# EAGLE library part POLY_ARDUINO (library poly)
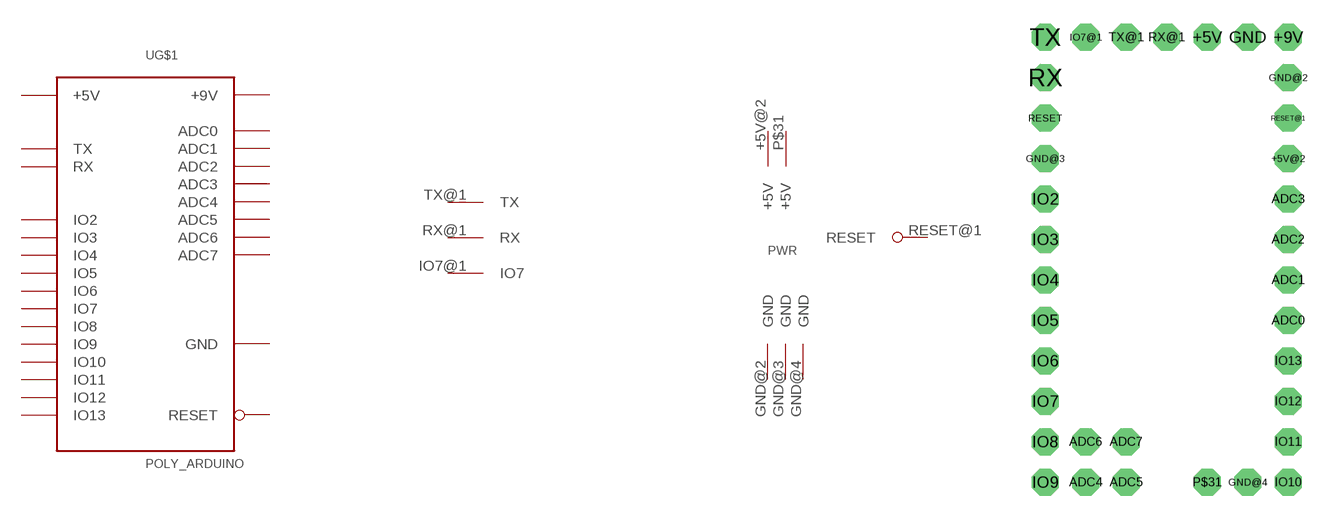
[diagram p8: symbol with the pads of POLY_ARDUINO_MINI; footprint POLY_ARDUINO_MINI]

Designator prefix -; gates G$1=POLY_ARDUINO G$2=POLY_ARDUINO_MINI_GND G$3=POLY_ARDUINO_MINI_OPT_IO

## POLY_ARDUINO  [POLY_ARDUINO_MINI]
+5V  G$1:+5V  pwr
+5V@2  G$2:+5V  pwr
+9V  G$1:+9V  pwr
ADC0  G$1:ADC0  in
ADC1  G$1:ADC1  in
ADC2  G$1:ADC2  in
ADC3  G$1:ADC3  in
ADC4  G$1:ADC4  in
ADC5  G$1:ADC5  in
ADC6  G$1:ADC6  in
ADC7  G$1:ADC7  in
GND  G$1:GND  sup
GND@2  G$2:GND  pwr
GND@3  G$2:GND  pwr
GND@4  G$2:GND  pwr
IO2  G$1:IO2
IO3  G$1:IO3
IO4  G$1:IO4
IO5  G$1:IO5
IO6  G$1:IO6
IO7  G$1:IO7
IO7@1  G$3:IO7
IO8  G$1:IO8
IO9  G$1:IO9
IO10  G$1:IO10
IO11  G$1:IO11
IO12  G$1:IO12
IO13  G$1:IO13
P$31  G$2:+5V  pwr
RESET  G$1:RESET
RESET@1  G$2:RESET  in
RX  G$1:RX  in
RX@1  G$3:RX  in
TX  G$1:TX  out
TX@1  G$3:TX  out

## Footprint POLY_ARDUINO_MINI (pad centres in mm)
drill 0.8 pad 1.676 octagon: +5V 11.43,29.21; +5V@2 16.51,21.59; +9V 16.51,29.21; ADC0 16.51,11.43; ADC1 16.51,13.97; ADC2 16.51,16.51; ADC3 16.51,19.05; ADC4 3.81,1.27; ADC5 6.35,1.27; ADC6 3.81,3.81; ADC7 6.35,3.81; GND 13.97,29.21; GND@2 16.51,26.67; GND@3 1.27,21.59; GND@4 13.97,1.27; IO2 1.27,19.05; IO3 1.27,16.51; IO4 1.27,13.97; IO5 1.27,11.43; IO6 1.27,8.89; IO7 1.27,6.35; IO7@1 3.81,29.21; IO8 1.27,3.81; IO9 1.27,1.27; IO10 16.51,1.27; IO11 16.51,3.81; IO12 16.51,6.35; IO13 16.51,8.89; P$31 11.43,1.27; RESET 1.27,24.13; RESET@1 16.51,24.13; RX 1.27,26.67; RX@1 8.89,29.21; TX 1.27,29.21; TX@1 6.35,29.21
